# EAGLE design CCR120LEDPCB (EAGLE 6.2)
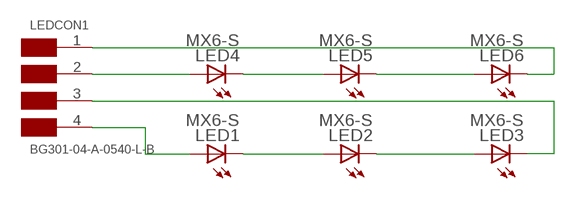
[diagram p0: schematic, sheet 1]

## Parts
LED1  MX6-S  [MX6-S]
LED2  MX6-S  [MX6-S]
LED3  MX6-S  [MX6-S]
LED4  MX6-S  [MX6-S]
LED5  MX6-S  [MX6-S]
LED6  MX6-S  [MX6-S]
LEDCON1  BG301-04-A-0540-L-B  [LEDCON_4_M]

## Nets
N$1: LED4.A LEDCON1.2
N$2: LED1.A LEDCON1.4
N$3: LED4.C LED5.A
N$4: LED5.C LED6.A
N$5: LED6.C LEDCON1.1
N$6: LED1.C LED2.A
N$7: LED2.C LED3.A
N$8: LED3.C LEDCON1.3

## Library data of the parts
LED1-LED6 = CCR_120VAC_LIB:MX6-S
LEDCON1 = CCR_120VAC_LIB:BG301-04-A-0540-L-B

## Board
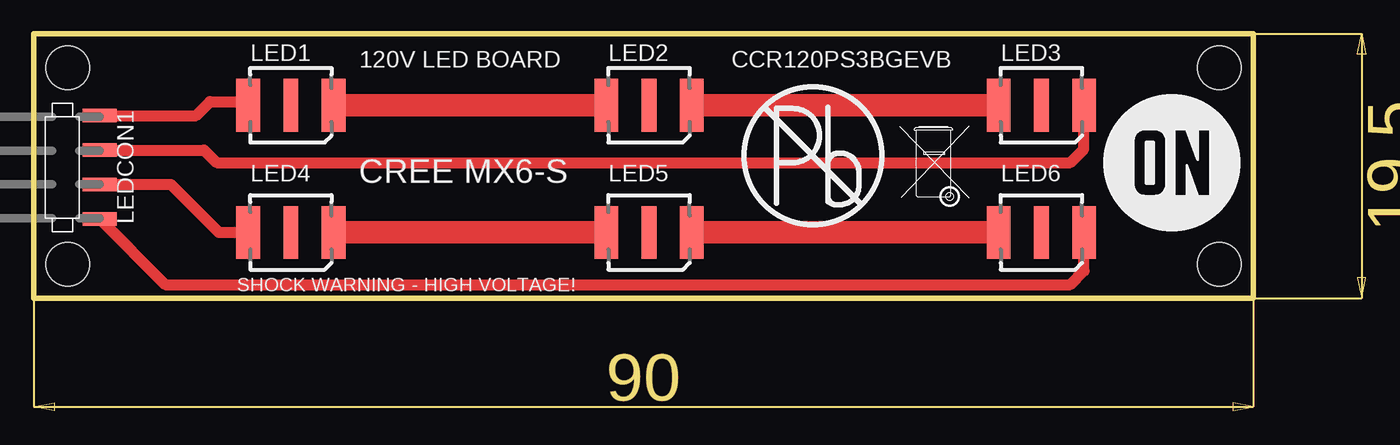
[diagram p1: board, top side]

Size 98.3 x 27.8 mm. Coordinates in mm from the lower left corner, seen from the top.
Outline: 0,8.3 0,27.8 90,27.8 90,8.3 0,8.3
Copper layers (1*16): Top 0.035mm / dielectric 1.5mm / Bottom 0.035mm
Design rules "default": minimum track width 10mil, minimum drill 24mil, track to track 8mil, track to pad 8mil, pad to pad 8mil, via to via 8mil, smd to smd 8mil, copper to edge 40mil, drill to drill 8mil, minimum pad ring 10mil, minimum via ring 8mil, stop-mask expansion 4mil, vias tented up to drill 0mil, thermal gap 10mil
Holes 3.2 mm at 2.5,25.3 2.5,10.8 87.5,25.3 87.5,10.8

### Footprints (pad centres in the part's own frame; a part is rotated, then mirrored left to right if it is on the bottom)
MX6-S = smd 1.75 x 3.9: A -3.15,0; C 3.15,0 | smd 1.1 x 3.9: P$1 0,0
LEDCON_4_M = smd 2.5 x 1: 1 0,2.54; 2 0,0; 3 0,-2.54; 4 0,-5.08

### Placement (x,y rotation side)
LED1  18.97,22.54 0 top
LED2  45.4,22.54 0 top
LED3  74.37,22.54 0 top
LED4  18.97,13.15 0 top
LED5  45.4,13.15 0 top
LED6  74.37,13.15 0 top
LEDCON1  4.85,16.69 180 top
U$1  [ON2]  84,18.3 0 top
U$2  [PB]  57.5,18.8 0 top
U$3  [BIN1]  66.5,18.3 0 top

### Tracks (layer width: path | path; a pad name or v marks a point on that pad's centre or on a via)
N$1
  Top 0.813: LEDCON1.2 10.11,16.69 13.65,13.15 LED4.A
N$2
  Top 0.813: LEDCON1.4 11.97,21.77 13,22.8 15.56,22.8 LED1.A
N$3
  Top 1.676: LED4.C LED5.A
N$4
  Top 1.676: LED5.C LED6.A
N$5
  Top 0.813: LEDCON1.1 9.7,9.3 76.5,9.3 77.52,10.32 LED6.C
N$6
  Top 1.676: LED1.C LED2.A
N$7
  Top 1.676: LED2.C LED3.A
N$8
  Top 0.813: LEDCON1.3 12.57,19.23 13.5,18.3 76.5,18.3 77.5,19.3 77.5,22.52 LED3.C

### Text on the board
tNames: 120V LED BOARD | CCR120PS3BGEVB | CREE MX6-S | SHOCK WARNING - HIGH VOLTAGE!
